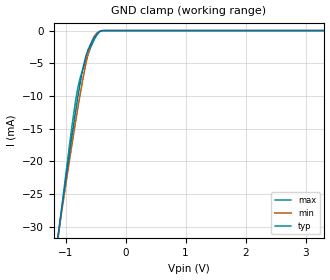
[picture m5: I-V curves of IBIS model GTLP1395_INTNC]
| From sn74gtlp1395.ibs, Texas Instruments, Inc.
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[Model]   GTLP1395_INTNC
Model_type  Input
Vinl = 0.8
Vinh = 2.0
| variable   typ   min   max
C_comp   2.76pF   1.90pF   3.89pF
[Temperature Range]   40   100   -40
| Ambient temperature   25   85   -40
[Voltage range]   3.3   3.15   3.45
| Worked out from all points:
|   GND clamp passes 1 mA (typ) near -0.51 V on its own axis
[GND Clamp]
| GTLP1395_INTNC
|   Voltage   I(typ)   I(min)   I(max)
-5.5V     -354.3mA   -327.1mA   -395.8mA
-1.15V    -33.04mA   -33.05mA   -33.71mA
-1.11V    -30.33mA   -30.56mA   -30.64mA
-890mV    -15.89mA   -17.25mA   -14.45mA
-835mV    -12.51mA   -14.09mA   -10.9mA
-795mV    -10.17mA   -11.85mA   -8.783mA
-695mV    -5.144mA   -6.648mA   -5.431mA
-610mV    -2.623mA   -3.059mA   -3.251mA
-545mV    -1.467mA   -1.304mA   -1.835mA
-460mV    -389.9uA   -251.6uA   -457.8uA
-365mV    -3.918uA   -10.79uA   -4.011uA
3.3V      166.6pA    582.9pA    1.325nA
